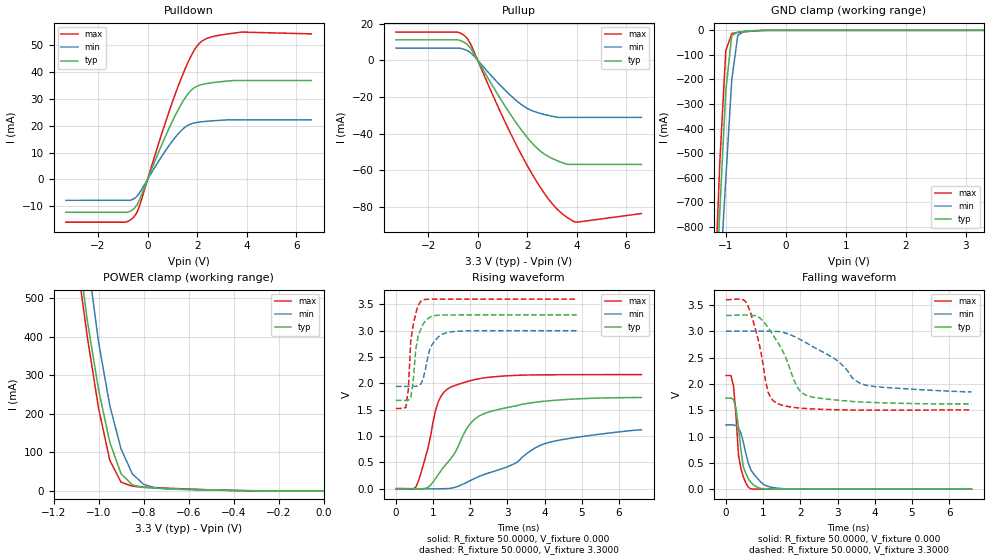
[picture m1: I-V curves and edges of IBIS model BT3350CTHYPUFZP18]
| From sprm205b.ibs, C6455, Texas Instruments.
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|   Model BT3350CTHYPUFZP18
[Model]   BT3350CTHYPUFZP18
Model_type   I/O
Polarity   Non-Inverting
Enable   Active-Low
Vinl =   0.8000V
Vinh =   2.0000V
Vmeas =   1.5000V
Cref =  10.0000pF
Rref =  50.0000
Vref =   1.5000V
C_comp   1.3673pF   1.3115pF   1.4386pF
[Temperature Range]   25.0000   0.1250k   -40.0000
[Pullup Reference]   3.3000V   3.0000V   3.6000V
[Pulldown Reference]   0.000V   0.000V   0.000V
[POWER Clamp Reference]   3.3000V   3.0000V   3.6000V
[GND Clamp Reference]   0.000V   0.000V   0.000V
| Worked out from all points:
|   slope of the pulldown table from 0 to 0.495 V, typ, clamps not added: 44 ohm
|   slope of the pullup table from 0 to 0.495 V, typ, clamps not added: 42.8 ohm
|   GND clamp passes 1 mA (typ) near -0.47 V on its own axis
|   POWER clamp passes 1 mA (typ) near -0.38 V on its own axis
|   rising waveform, R_fixture 50.0000, V_fixture 0.000: 20-80 % time 1.04ns typ, 1.99ns min, 468ps max; typ from 0 V to 1.73 V
|   rising waveform, R_fixture 50.0000, V_fixture 3.3000: 20-80 % time 183ps typ, 274ps min, 151ps max; typ from 1.68 V to 3.3 V
|   falling waveform, R_fixture 50.0000, V_fixture 0.000: 20-80 % time 210ps typ, 368ps min, 161ps max; typ from 1.73 V to 0 V
|   falling waveform, R_fixture 50.0000, V_fixture 3.3000: 20-80 % time 675ps typ, 1.27ns min, 371ps max; typ from 3.3 V to 1.62 V
[Pulldown]
| voltage   I(typ)   I(min)   I(max)
-3.3V     -12.32mA   -7.84mA    -16.01mA
-800mV    -12.32mA   NA         -15.72mA
-500mV    -10.49mA   -6.966mA   -13.46mA
-300mV    -7.034mA   -4.709mA   -9.192mA
600mV     13.53mA    9.001mA    17.88mA
1.3V      27.11mA    17.65mA    36.39mA
1.8V      33.62mA    20.84mA    46.89mA
2V        34.78mA    21.25mA    49.84mA
2.2V      35.39mA    21.5mA     51.66mA
2.6V      36.06mA    21.83mA    53.22mA
3.5V      36.9mA     NA         54.62mA
6.6V      36.9mA     22.21mA    54.31mA
[Pullup]
| voltage   I(typ)   I(min)   I(max)
-3.3V     11.22mA    6.704mA    15.43mA
-800mV    11.22mA    6.703mA    15.43mA
-500mV    9.447mA    5.764mA    13.06mA
-300mV    6.8mA      4.287mA    9.245mA
1V        -22.82mA   -14.89mA   -30.69mA
2V        -42.2mA    -26.29mA   -57.53mA
2.4V      -48.09mA   -28.51mA   -66.74mA
2.8V      -52.14mA   -29.95mA   -74.81mA
3.2V      -54.81mA   -31.05mA   -81.26mA
3.5V      -56.33mA   NA         -84.78mA
3.7V      -56.86mA   NA         -86.64mA
6.6V      -56.86mA   -31.2mA    -83.72mA
[GND_clamp]
| voltage   I(typ)   I(min)   I(max)
-3.3V     -15.87A    -14.34A    -17.08A
-1.2V     -1.264A    -1.454A    -1.162A
-1.1V     -739.5mA   -1.022A    -539.8mA
-1V       -245.2mA   -606mA     -83.29mA
-900mV    -21.28mA   -200.9mA   -12.95mA
-800mV    -6.934mA   -20.53mA   -8.836mA
-700mV    -4.617mA   -4.425mA   -6.307mA
-300mV    -39.21uA   -55.39uA   -61.04uA
3.3V      64.31uA    87.36uA    295.9nA
[POWER_clamp]
| voltage   I(typ)   I(min)   I(max)
-3.3V     13.83A     12.48A     14.95A
-1.1V     665.8mA    853.9mA    613.9mA
-1.05V    441.8mA    607.3mA    399.6mA
-1V       262.7mA    385.8mA    214.7mA
-950mV    126.2mA    221.3mA    79.62mA
-900mV    44.66mA    108.9mA    22.72mA
-850mV    15.65mA    44.49mA    12.15mA
-800mV    8.944mA    17.22mA    9.922mA
-750mV    7.042mA    8.262mA    8.555mA
-650mV    5.002mA    4.149mA    6.078mA
-350mV    702.5uA    800.3uA    625.3uA
0V        112.6nA    175nA      370.7nA
[Ramp]
| variable   typ   min   max
dV/dt_r   1.0385/1.0250n   0.6701/2.0375n   1.3000/0.4628n
dV/dt_f   1.0079/0.6682n   0.6918/1.3279n   1.2563/0.3674n
R_load = 50.0000
[Rising Waveform]
R_fixture = 50.0000
V_fixture = 0.000
V_fixture_min = 0.000
V_fixture_max = 0.000
| time   V(typ)   V(min)   V(max)
0s        38.02uV    34.08uV    68.16uV
533.3ps   -7.268mV   -8.356uV   27.93mV
866.7ps   27.6mV     -3.094mV   786.6mV
1.133ns   261.4mV    -3.207mV   1.639V
1.467ns   563.3mV    7.032mV    1.924V
2ns       1.235V     153mV      2.05V
2.467ns   1.449V     292mV      2.112V
3.2ns     1.569V     479.4mV    2.15V
4.067ns   1.665V     868.9mV    2.162V
6.6ns     1.731V     1.117V     2.167V
[Rising Waveform]
R_fixture = 50.0000
V_fixture = 3.3000
V_fixture_min = 3.0000
V_fixture_max = 3.6000
| time   V(typ)   V(min)   V(max)
0s        1.676V     1.942V     1.523V
266.7ps   1.677V     1.943V     1.541V
333.3ps   1.678V     1.943V     1.883V
400ps     1.733V     1.943V     2.815V
466.7ps   2.059V     1.943V     3.117V
533.3ps   2.643V     1.943V     3.33V
666.7ps   3.025V     1.983V     3.559V
933.3ps   3.262V     2.695V     3.598V
1.333ns   3.297V     2.955V     3.599V
4.867ns   3.3V       3V         3.6V
|  4.9333nS   3.2999V   2.9998V   3.6000V
|  5.0000nS   3.2999V   2.9998V   3.6000V
|  5.0667nS   3.2999V   2.9998V   3.6000V
|  5.1333nS   3.2999V   2.9998V   3.6000V
|  5.2000nS   3.2999V   2.9998V   3.6000V
|  5.2667nS   3.2999V   2.9998V   3.6000V
|  5.3333nS   3.2999V   2.9998V   3.6000V
|  5.4000nS   3.2999V   2.9998V   3.6000V
|  5.4667nS   3.2999V   2.9998V   3.6000V
|  5.5333nS   3.2999V   2.9998V   3.6000V
|  5.6000nS   3.2999V   2.9998V   3.6000V
|  5.6667nS   3.2999V   2.9998V   3.6000V
|  5.7333nS   3.2999V   2.9998V   3.6000V
|  5.8000nS   3.2999V   2.9998V   3.6000V
|  5.8667nS   3.2999V   2.9998V   3.6000V
|  5.9333nS   3.3000V   2.9998V   3.6000V
|  6.0000nS   3.3000V   2.9998V   3.6000V
|  6.0667nS   3.3000V   2.9998V   3.6000V
|  6.1333nS   3.3000V   2.9999V   3.6000V
|  6.2000nS   3.3000V   2.9999V   3.6000V
|  6.2667nS   3.3000V   2.9999V   3.6000V
|  6.3333nS   3.3000V   2.9999V   3.6000V
|  6.4000nS   3.3000V   2.9999V   3.6000V
|  6.4667nS   3.3000V   2.9999V   3.6000V
|  6.6000nS   3.3000V   2.9999V   3.6000V
[Falling Waveform]
R_fixture = 50.0000
V_fixture = 0.000
V_fixture_min = 0.000
V_fixture_max = 0.000
| time   V(typ)   V(min)   V(max)
0s        1.728V     1.22V      2.16V
133.3ps   1.729V     1.22V      2.158V
200ps     1.704V     1.22V      1.967V
333.3ps   1.173V     1.164V     656.1mV
400ps     739.4mV    1.065V     389mV
466.7ps   415.1mV    886.9mV    230.3mV
666.7ps   128.2mV    370.5mV    6.445mV
1ns       6.015mV    96.02mV    706.6uV
1.467ns   648.1uV    14.07mV    292.3uV
6.6ns     7.674uV    73.87uV    23.34uV
[Falling Waveform]
R_fixture = 50.0000
V_fixture = 3.3000
V_fixture_min = 3.0000
V_fixture_max = 3.6000
| time   V(typ)   V(min)   V(max)
0s        3.3V       3V         3.6V
533.3ps   3.307V     3.005V     3.558V
866.7ps   3.275V     3.005V     2.836V
1.133ns   3.066V     3.001V     1.839V
1.4ns     2.777V     2.995V     1.623V
1.933ns   1.919V     2.867V     1.544V
2.2ns     1.772V     2.763V     1.529V
2.933ns   1.695V     2.472V     1.511V
3.733ns   1.653V     1.981V     1.502V
6.6ns     1.62V      1.847V     1.506V
